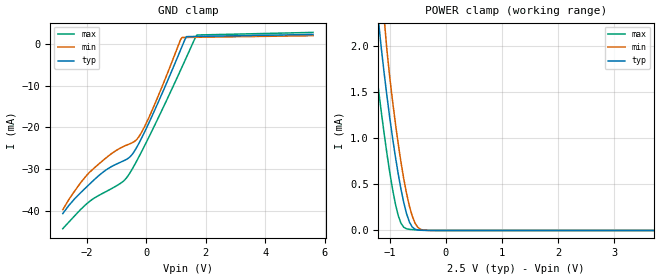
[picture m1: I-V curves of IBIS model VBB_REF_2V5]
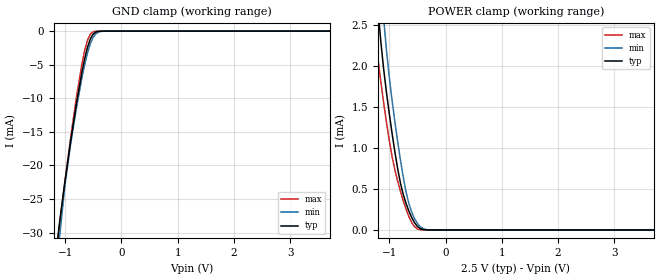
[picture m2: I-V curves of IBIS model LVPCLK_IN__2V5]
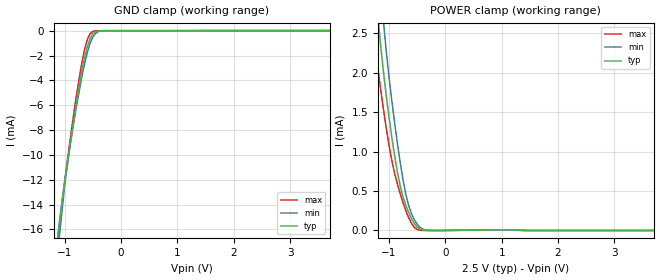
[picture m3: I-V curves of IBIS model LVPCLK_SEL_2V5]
| IBIS file CDCLVP110 for Texas Instruments Version 2.5V and 3.3V
[IBIS ver]   3.2
[File name]   cdclvp110.ibs
[File Rev]   2.0
[Date]   March 22th 2004
[Source]   File originated at Texas Instruments Incorporated.
   HPA HIGH SPEED COMMUNICATION AND CONTROLL, HSCC.
|REVISON LOG: 2.0 3/22/2004 new IBIS models for 2.5V and 3.3V VCC range.
|   Combined both VCC ranges to one IBIS file with 3.3V VCC
|   as the default VCC setting.
|   Drive current and differential output voltage vs frequency
|   was correlated to real silicon. In the IBIS simulation, Tf
|   turns out to be about 10%-15% faster as measurements on real
|   silicon. This was kept unchanged to keep crosspoint at about
|   common mode voltage.
|   The non-montonic Warnings are due to input current
|   characteristic of the SEL input.
[Notes]
[Disclaimer]
(C) Copyright Texas Instruments Incorporated 2004
   All rights reserved
  Texas Instruments Incorporated hereby grants the user of this IBIS
model a non-exclusive, nontransferable license to use this IBIS model
under the following terms.  Before using this IBIS model, the user
should read this license.  If the user does not accept these terms,
the IBIS model should be returned to Texas Instruments within 30 days.
  The user is granted this license only to use the IBIS model and
is not granted rights to sell, load, rent, lease or license the IBIS
model in whole or in part, or in modified form to anyone other than
user.  User may modify the IBIS model to suit its specific applications
but rights to derivative works and such modifications shall belong to
Texas Instruments.
  This IBIS model is provided on an "AS IS" basis and Texas Instruments
makes absolutely no warranty with respect to the information contained
herein.  TEXAS INSTRUMENTS DISCLAIMS AND CUSTOMER WAIVES ALL WARRANTIES,
EXPRESS OR IMPLIED, INCLUDING WARRANTIES OF MERCHANTABILITY OR FITNESS
FOR A PARTICULAR PURPOSE. The entire risk as to quality and performance
is with the Customer. ACCORDINGLY, IN NO EVENT SHALL THE COMPANY BE LIABLE
FOR ANY DAMAGES, WHETHER IN CONTRACT OR TORT,INCLUDING ANY LOST PROFITS
OR OTHER INCIDENTAL, CONSEQUENTIAL, EXEMPLARY, OR PUNITIVE DAMAGES ARISING
OUT OF THE USE OR APPLICATION OF THE IBIS model provided in this package.
Further, Texas Instruments reserves the right to discontinue or make changes
without notice to any product herein to improve reliability, function, or
design. Texas Instruments does not convey any license under patent rights
or any other intellectual property rights, including those of third parties.
Contact Texas Instruments at ATTN: HPA-High Speed Communication & Control, HSC
|   Component CDCLVP110
[Copyright]   Copyright 2004, Texas Instruments, All Rights Reserved
[Component]   CDCLVP110
[Manufacturer]  Texas Instruments Incorporated
[Package]
|   typ   min   max
R_pkg   0.1026   0.0423   0.1248
L_pkg   3.424nH   2.117nH   4.030nH
C_pkg   0.276pF   0.217pF   0.610pF
[Pin] signal_name  model_name  R_pin  L_pin  C_pin
1  VCC   POWER   0.0621   2.572nH   0.422pF
2  CLK_SEL   LVPCLK_SEL   0.1106   3.670nH   0.268pF
3  CLK0_T   LVPCLK_IN   0.1043   3.429nH   0.235pF
4  CLK0_N   LVPCLK_IN   0.1018   3.304nH   0.218pF
5  VBB   VBB_REF   0.1022   3.313nH   0.218pF
6  CLK1_T   LVPCLK_IN   0.1054   3.453nH   0.228pF
7  CLK1_N   LVPCLK_IN   0.1129   3.696nH   0.247pF
8  VEE   POWER   0.0621   2.573nH   0.514pF
9  VCC   POWER   0.0621   2.572nH   0.422pF
10 Q9B   LVPCLK_OUT   0.1132   3.725nH   0.261pF
11 Q9   LVPCLK_OUT   0.1072   3.492nH   0.235pF
12 Q8B   LVPCLK_OUT   0.1048   3.371nH   0.219pF
13 Q8   LVPCLK_OUT   0.1053   3.380nH   0.221pF
14 Q7B   LVPCLK_OUT   0.1083   3.516nH   0.230pF
15 Q7   LVPCLK_OUT   0.1148   3.750nH   0.253pF
16 VCC   POWER   0.0621   2.572nH   0.422pF
17 Q6B   LVPCLK_OUT   0.1235   3.997nH   0.288pF
18 Q6   LVPCLK_OUT   0.1116   3.673nH   0.265pF
19 Q5B   LVPCLK_OUT   0.1048   3.439nH   0.234pF
20 Q5   LVPCLK_OUT   0.1020   3.309nH   0.219pF
21 Q4B   LVPCLK_OUT   0.1020   3.308nH   0.217pF
22 Q4   LVPCLK_OUT   0.1047   3.440nH   0.227pF
23 Q3B   LVPCLK_OUT   0.1115   3.690nH   0.250pF
24 Q3   LVPCLK_OUT   0.1232   3.995nH   0.284pF
25 VCC   POWER   0.0621   2.572nH   0.422pF
26 Q2B   LVPCLK_OUT   0.1151   3.751nH   0.258pF
27 Q2   LVPCLK_OUT   0.1082   3.517nH   0.236pF
28 Q1B   LVPCLK_OUT   0.1052   3.381nH   0.219pF
29 Q1   LVPCLK_OUT   0.1048   3.371nH   0.219pF
30 Q0B   LVPCLK_OUT   0.1071   3.493nH   0.227pF
31 Q0   LVPCLK_OUT   0.1131   3.728nH   0.256pF
32 VCC   POWER   0.0621   2.572nH   0.422pF
[Diff_Pin]  inv_pin  vdiff   tdelay_typ  tdelay_min  tdelay_max
| The '+' pin is   Diff_pin,   the '-' pin is the   Inv_pin
| Receiver Pins  |  Receiver Vth = +/-200mV
3   4   0.2   0ns   0ns   0ns   | CLK0_T /_N
6   7   0.2   0ns   0ns   0ns   | CLK1_T /_N
| Driver Pins   |  Rload = 50 OHM to VCC-2 termination
31   30   NA   0ns   0ns   0ns   | Y0 / Y0-
29   28   NA   0ns   0ns   0ns   | Y1 / Y1-
27   26   NA   0ns   0ns   0ns   | Y2 / Y2-
24   23   NA   0ns   0ns   0ns   | Y3 / Y3-
22   21   NA   0ns   0ns   0ns   | Y4 / Y4-
20   19   NA   0ns   0ns   0ns   | Y5 / Y5-
18   17   NA   0ns   0ns   0ns   | Y6 / Y6-
15   14   NA   0ns   0ns   0ns   | Y7 / Y7-
13   12   NA   0ns   0ns   0ns   | Y8 / Y8-
11   10   NA   0ns   0ns   0ns   | Y9 / Y9-
[Model Selector]   LVPCLK_SEL
LVPCLK_SEL_3V3  MODEL for VDD= 3.0V - 3.8V
LVPCLK_SEL_2V5  MODEL for VDD= 2.375V - 2.75V
[Model Selector]   LVPCLK_IN
LVPCLK_IN__3V3  MODEL for VDD= 3.0V - 3.8V
LVPCLK_IN__2V5  MODEL for VDD= 2.375V - 2.75V
[Model Selector]   LVPCLK_OUT
LVPCLK_OUT_3V3  MODEL for VDD= 3.0V - 3.8V
LVPCLK_OUT_2V5  MODEL for VDD= 2.375V - 2.75V
[Model Selector]   VBB_REF
VBB_REF_3V3  MODEL for VDD= 3.0V - 3.8V
VBB_REF_2V5  MODEL for VDD= 2.375V - 2.75V
| Models and submodels in the file (8): VBB_REF_2V5 (Terminator), LVPCLK_IN__2V5 (Input), LVPCLK_SEL_2V5 (Input), LVPCLK_OUT_2V5 (3-state_ECL), VBB_REF_3V3 (Terminator), LVPCLK_IN__3V3 (Input), LVPCLK_SEL_3V3 (Input), LVPCLK_OUT_3V3 (3-state_ECL)
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|   Reference Voltage Model for 2.5V VCC range   |
[Model]   VBB_REF_2V5
Model_type   Terminator
| Signals   VBB
| variable   typ   min   max
C_comp   0.5pF   NA   NA
[Temperature Range]   40C   110C   -40C
[Voltage range]   2.5V   2.375V   2.75V
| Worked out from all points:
|   POWER clamp passes 1 mA (typ) near -0.95 V on its own axis
[POWER Clamp]
|   40C:2.5V:nominal  110C:2.375V:weak  -40C:2.75V:strong
|  Voltage   I(typ)   I(min)   I(max)
-2.8V     44.65mA    68.92mA    23.89mA
-1.35V    3.669mA    5.59mA     2.325mA
-1.3V     3.09mA     4.776mA    2.049mA
-1.2V     2.273mA    3.336mA    1.53mA
-1.1V     1.711mA    2.309mA    1.054mA
-1.05V    1.461mA    1.957mA    835.4uA
-900mV    803.8uA    1.168mA    291.6uA
-800mV    449.9uA    742.7uA    79.27uA
-700mV    181.8uA    401.2uA    18.13uA
-550mV    13.65uA    80.74uA    7.566uA
-400mV    1.235uA    4.022uA    3.439uA
5.6V      0A         0A         0A
[GND Clamp]
|   40C:2.5V:nominal  110C:2.375V:weak  -40C:2.75V:strong
|  Voltage   I(typ)   I(min)   I(max)
-2.8V     -40.6mA    -39.67mA   -44.2mA
-2.4V     -37.04mA   -35.18mA   -41.12mA
-1.9V     -33.55mA   -30.73mA   -37.68mA
-1.4V     -30.44mA   -27.6mA    -35.54mA
-800mV    -28.13mA   -24.7mA    -33.06mA
-450mV    -26.26mA   -23.61mA   -29.72mA
-250mV    -23.87mA   -22.27mA   -27.1mA
50mV      -19.54mA   -18.27mA   -22.91mA
1.2V      -705.4uA   1.46mA     -5.607mA
1.35V     1.677mA    1.48mA     -3.256mA
1.7V      1.726mA    1.521mA    2.064mA
5.6V      2.195mA    1.906mA    2.688mA
|   Diff. Receiver Input Model for 2.5V VCC range   |
[Model]   LVPCLK_IN__2V5
Model_type   Input
| Signals   CLK0_T, CLK1_T,CLK0_N, CLK1_N
| variable   typ   min   max
C_comp   0.5pF   NA   NA
| Vicm(typ)=(VCC-0.3V-1V)=2.500V-1.3V=1.200V/2+1V ==>1.6000V +/-0.25V
| Vicm(min)=(+1V) ==> 1.25V +/-0.25V
| Vicm(max)=(VCC-0.3V)=2.450V ==> 2.20V +/-0.25V
Vinl = 1.35V   |
Vinh = 1.85V   |
[Model Spec]
|   VCC=2.5V   VCC=2.375V   VCC=2.75V
Vinl   1.35V   1.00V   1.95V
Vinh   1.85V   1.50V   2.45V
[Temperature Range]   40C   110C   -40C
[Voltage range]   2.5V   2.375V   2.75V
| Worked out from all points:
|   GND clamp passes 1 mA (typ) near -0.54 V on its own axis
|   POWER clamp passes 1 mA (typ) near -0.91 V on its own axis
[POWER Clamp]
|   40C:2.5V:nominal  110C:2.375V:weak  -40C:2.75V:strong
|  Voltage   I(typ)   I(min)   I(max)
-2.8V     48.73mA    76.99mA    23.41mA
-1.25V    3.146mA    4.079mA    2.413mA
-1.2V     2.693mA    3.533mA    2.089mA
-1.15V    2.3mA      3.03mA     1.811mA
-1.1V     1.967mA    2.582mA    1.557mA
-1.05V    1.68mA     2.197mA    1.317mA
-950mV    1.179mA    1.582mA    895.9uA
-800mV    568.8uA    847.8uA    469uA
-650mV    228.5uA    318.7uA    161uA
-500mV    43.24uA    80.19uA    12.52uA
-250mV    56.05nA    514.5nA    1.202nA
5.6V      -454.4pA   -13.13nA   -471.7pA
[GND Clamp]
|   40C:2.5V:nominal  110C:2.375V:weak  -40C:2.75V:strong
|  Voltage   I(typ)   I(min)   I(max)
-2.8V     -270.3mA   -305.8mA   -238.1mA
-1.2V     -36.15mA   -42.21mA   -35.95mA
-1.1V     -28.63mA   -30.86mA   -28.94mA
-1V       -22.25mA   -22.78mA   -22.21mA
-900mV    -16.35mA   -16.78mA   -15.83mA
-800mV    -10.9mA    -11.56mA   -9.953mA
-700mV    -6.1mA     -6.953mA   -4.88mA
-600mV    -2.375mA   -3.219mA   -1.316mA
-500mV    -439.4uA   -906.1uA   -101.6uA
-400mV    -35.43uA   -131.9uA   -2.723uA
-250mV    -349.7nA   -3.494uA   -4.457nA
5.6V      880.3pA    17.67nA    448.2pA
|   Clock Select Input  Model for 2.5V VCC range   |
[Model]   LVPCLK_SEL_2V5
Model_type   Input
| Signals   CLK_SEL
| variable   typ   min   max
C_comp   0.5pF   NA   NA
Vinl = 1.025V   | VCC-1.475 (max)
Vinh = 1.335V   | VCC-1.165 (min)
[Model Spec]
|   VCC=2.5V   VCC=2.375V   VCC=2.75V
Vinl   1.025V   0.90V   1.275V
Vinh   1.335V   1.21V   1.585V
[Temperature Range]   40C   110C   -40C
[Voltage range]   2.5V   2.375V   2.75V
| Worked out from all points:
|   GND clamp passes 1 mA (typ) near -0.58 V on its own axis
|   POWER clamp passes 1 mA (typ) near -0.91 V on its own axis
[POWER Clamp]
|   40C:2.5V:nominal  110C:2.375V:weak  -40C:2.75V:strong
|  Voltage   I(typ)   I(min)   I(max)
-2.8V     48.3mA     76.31mA    23.2mA
-1.3V     3.667mA    4.675mA    2.799mA
-1.2V     2.747mA    3.583mA    2.082mA
-1.15V    2.36mA     3.097mA    1.799mA
-1.1V     2.021mA    2.663mA    1.544mA
-1.05V    1.719mA    2.284mA    1.306mA
-950mV    1.184mA    1.647mA    887.9uA
-800mV    563.8uA    857.8uA    464.8uA
-650mV    226.4uA    316uA      159.5uA
-500mV    42.85uA    79.46uA    12.41uA
-250mV    55.18nA    506.4nA    797.7pA
5.6V      -454.4pA   -13.13nA   -471.7pA
[GND Clamp]
|   40C:2.5V:nominal  110C:2.375V:weak  -40C:2.75V:strong
|  Voltage   I(typ)   I(min)   I(max)
-2.8V     -146.8mA   -166.1mA   -129.4mA
-1.2V     -19.64mA   -22.93mA   -19.53mA
-1.1V     -15.55mA   -16.76mA   -15.72mA
-1V       -12.09mA   -12.38mA   -12.06mA
-900mV    -8.882mA   -9.114mA   -8.599mA
-800mV    -5.924mA   -6.282mA   -5.407mA
-700mV    -3.314mA   -3.777mA   -2.651mA
-600mV    -1.29mA    -1.749mA   -715uA
-500mV    -238.7uA   -492.2uA   -55.21uA
-400mV    -19.24uA   -71.63uA   -1.479uA
-250mV    -190.1nA   -1.9uA     -2.514nA
5.6V      6.936uA    5.361uA    9.426uA
